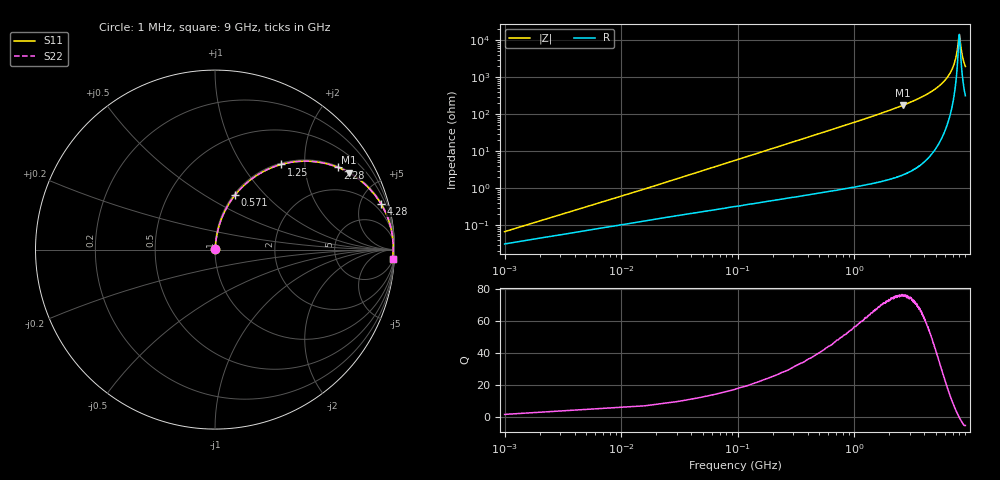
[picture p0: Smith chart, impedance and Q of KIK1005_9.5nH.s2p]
!version-3
!date-01.2023
!Series
# MHz S RI R 50
!Freq ReS11 ImS11 ReS21 ImS21 ReS12 ImS12 ReS22 ImS22
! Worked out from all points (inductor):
!   601 points, 1 MHz to 9 GHz, reference 50 ohm
!   read as one part in series: L = 9.5 nH near 46 MHz
!   highest Q = 76.2 at 2.6 GHz (marker M1), where L = 10.6 nH
!   self-resonance near 7.97 GHz
!   S11 on the Smith chart (normalised r, x): 1 MHz: 1.00, +0.00; 571 MHz: 1.02, +0.69; 1.25 GHz: 1.02, +1.52; 2.28 GHz: 1.04, +2.97; 4.28 GHz: 1.13, +7.16; 9 GHz: 7, -38
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1  0.00033 0.000597  0.9997 -0.000597  0.9997 -0.000597  0.00033 0.000597
61  0.00388 0.0362  0.9961 -0.0362  0.9961 -0.0362  0.00388 0.0362
91  0.00605 0.0538  0.9939 -0.0538  0.9939 -0.0538  0.00605 0.0538
121  0.00875 0.0713  0.9912 -0.0713  0.9912 -0.0713  0.00875 0.0713
196  0.0179 0.1144  0.9821 -0.1144  0.9821 -0.1144  0.0179 0.1144
286  0.0335 0.1643  0.9665 -0.1643  0.9665 -0.1643  0.0335 0.1643
571  0.1106 0.3023  0.8894 -0.3023  0.8894 -0.3023  0.1106 0.3023
1250  0.3696 0.4747  0.6304 -0.4747  0.6304 -0.4747  0.3696 0.4747
1520  0.469 0.4916  0.531 -0.4916  0.531 -0.4916  0.469 0.4916
2280  0.6851 0.4579  0.3149 -0.4579  0.3149 -0.4579  0.6851 0.4579
2600  0.7474 0.428  0.2526 -0.428  0.2526 -0.428  0.7474 0.428
3020  0.812 0.3841  0.188 -0.3841  0.188 -0.3841  0.812 0.3841
4280  0.9238 0.2566  0.0762 -0.2566  0.0762 -0.2566  0.9238 0.2566
4520  0.9362 0.2348  0.0638 -0.2348  0.0638 -0.2348  0.9362 0.2348
6020  0.9808 0.1172  0.0192 -0.1172  0.0192 -0.1172  0.9808 0.1172
6950  0.9908 0.0575  0.00922 -0.0575  0.00922 -0.0575  0.9908 0.0575
7520  0.9929 0.0248  0.00705 -0.0248  0.00705 -0.0248  0.9929 0.0248
7700  0.9931 0.015  0.00685 -0.015  0.00685 -0.015  0.9931 0.015
7920  0.9931 0.00303  0.00689 -0.00303  0.00689 -0.00303  0.9931 0.00303
8000  0.993 -0.000871  0.00697 0.000871  0.00697 0.000871  0.993 -0.000871
8430  0.992 -0.0228  0.00802 0.0228  0.00802 0.0228  0.992 -0.0228
9000  0.9892 -0.0497  0.0107 0.0497  0.0107 0.0497  0.9892 -0.0497
